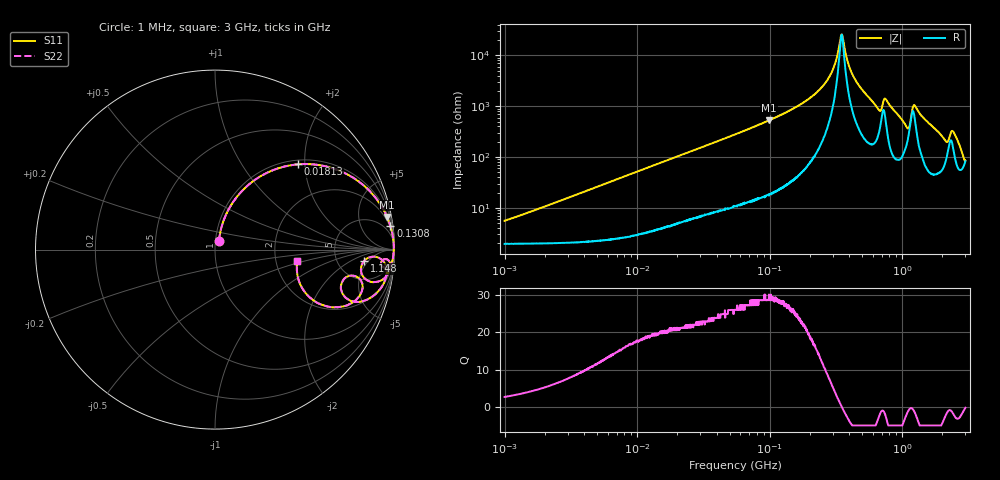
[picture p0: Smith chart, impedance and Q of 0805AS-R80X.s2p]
!s-Parameter Generated by FASTRON Sdn. Bhd.
!FASTRON P/N : 0805AS-R80X
!Keysight Technologies: E4991B_MY54100416_A.01.15
!Date: Mon Jun 15 12:56:07 2026
!Version  :Rev01  Mon Jun 15 12:56:07 2026
!Data & Calibration Information:
!Freq  S11  S21  S12  S22
!PortZ  Port1:50+j0  Port2:50+j0
!When reading reference impedance value at option line is always used.
! Remarks : This data is being provided solely for informational purposes.
# Hz S dB R 50
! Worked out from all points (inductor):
!   1601 points, 1 MHz to 3 GHz, reference 50 ohm
!   read as one part in series: L = 826 nH near 1.133 MHz
!   highest Q = 28.7 at 98.85 MHz (marker M1), where L = 844 nH
!   self-resonance near 348.9 MHz
!   S11 on the Smith chart (normalised r, x): 1 MHz: 1.04, +0.10; 18.13 MHz: 1.09, +1.85; 130.8 MHz: 2, +15; 1.148 GHz: 9, -4; 3 GHz: 2.65, -0.43
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1000000  -25.30 66.5  -0.18 -2.9  -0.18 -2.9  -25.30 66.5
3804036  -14.40 72.9  -0.34 -10.9  -0.34 -10.9  -14.40 72.9
1.447069e7  -4.69 51.5  -2.12 -35.6  -2.12 -35.6  -4.69 51.5
1.812522e7  -3.55 45.7  -2.90 -41.6  -2.90 -41.6  -3.55 45.7
5.504702e7  -0.63 19.4  -9.57 -68.4  -9.57 -68.4  -0.63 19.4
9.885493e7  -0.21 10.7  -14.60 -77.4  -14.60 -77.4  -0.21 10.7
1.308271e8  -0.12 7.6  -17.50 -80.3  -17.50 -80.3  -0.12 7.6
2.083556e8  -0.05 3.7  -23.90 -83.2  -23.90 -83.2  -0.05 3.7
2.870054e8  -0.03 1.4  -32.40 -80.3  -32.40 -80.3  -0.03 1.4
3.50605e8  -0.03 -0.0  -48.30 2.0  -48.30 2.0  -0.03 -0.0
4.0536e8  -0.04 -1.0  -34.60 75.5  -34.60 75.5  -0.04 -1.0
4.75755e8  -0.05 -2.3  -28.00 80.0  -28.00 80.0  -0.05 -2.3
6.652545e8  -0.38 -6.0  -19.00 64.3  -19.00 64.3  -0.38 -6.0
7.42674e8  -0.29 -3.5  -23.30 59.6  -23.30 59.6  -0.29 -3.5
7.925923e8  -0.17 -5.0  -21.10 74.9  -21.10 74.9  -0.17 -5.0
1.070143e9  -0.97 -11.7  -13.20 55.5  -13.20 55.5  -0.97 -11.7
1.147801e9  -1.58 -4.3  -14.90 20.4  -14.90 20.4  -1.58 -4.3
1.249715e9  -0.46 -4.6  -20.60 54.4  -20.60 54.4  -0.46 -4.6
2.061253e9  -1.54 -20.4  -8.82 53.6  -8.82 53.6  -1.54 -20.4
2.492946e9  -1.42 -16.5  -10.30 52.4  -10.30 52.4  -1.42 -16.5
2.75535e9  -2.84 -26.4  -6.43 42.1  -6.43 42.1  -2.84 -26.4
3e9  -6.67 -7.8  -5.29 6.7  -5.29 6.7  -6.67 -7.8
